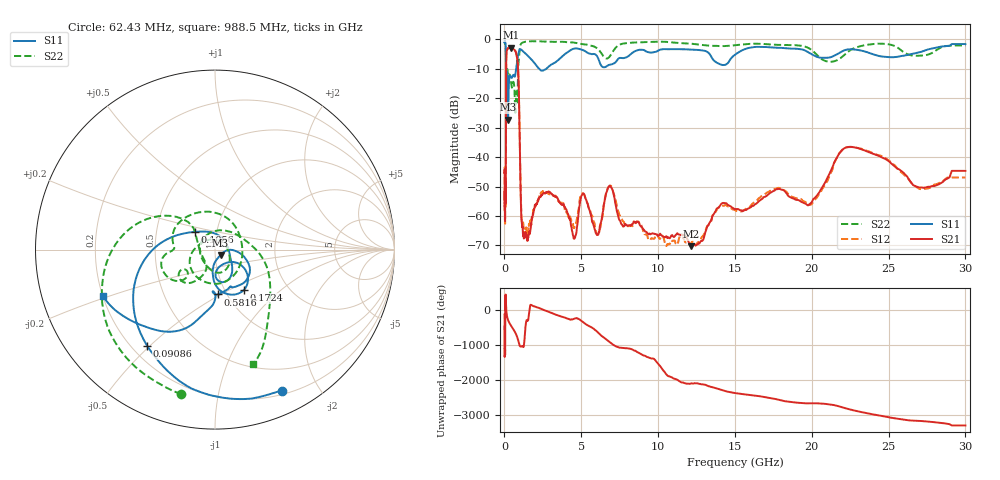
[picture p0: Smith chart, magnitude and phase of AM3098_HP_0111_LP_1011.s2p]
! Date/Time: Thu, Feb 28, 2019 8:39 AM
! Network Analyzer: Agilent Technologies E8364B Rev: A.07.50.67
! Sweep from 0.010 to 30.000 GHz, 1601 Points, Sweep Type: LOG
! Power Supply: 5.022 V, 0.002 A
# Hz S DB R 50
!freq MagS11 AngS11 MagS21 AngS21 MagS12 AngS12 MagS22 AngS22
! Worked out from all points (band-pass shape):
!   1601 points, 10 MHz to 30 GHz, reference 50 ohm
!   highest |S21| = -2.83 dB at 409.7 MHz (marker M1); lowest = -70.2 dB at 12.13 GHz (marker M2)
!   |S21| within 3 dB of the highest: 122.1 MHz to 807.7 MHz (685.6 MHz wide, 147 % of centre)
!   lowest |S11| = -27.2 dB at 238.7 MHz (marker M3), VSWR 1.09, Z = 53.1 - j3.22 ohm
!   |S11| at or under -10 dB: 102.2 MHz to 756.9 MHz (654.8 MHz wide, 152 % of centre); 2.273 GHz to 2.717 GHz (444.2 MHz wide, 17.8 % of centre)
!   |S22| runs from -24.9 to -0.6 dB; largest |S21 - S12| = 0.012
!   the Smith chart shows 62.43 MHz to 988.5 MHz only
!   S11 on the Smith chart (normalised r, x): 62.43 MHz: 0.24, -1.56; 90.86 MHz: 0.26, -0.49; 105.6 MHz: 0.78, +0.16; 172.4 MHz: 1.22, -0.60; 581.6 MHz: 0.91, -0.48; 988.5 MHz: 0.20, -0.19
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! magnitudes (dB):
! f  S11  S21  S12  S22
! 10 MHz  -0.4  -45.3  -43.3  -0.6
! 38.04 MHz  -0.4  -61.4  -60.0  -0.9
! 62.43 MHz  -1.2  -51.6  -51.8  -1.7
! 90.86 MHz  -3.7  -43.3  -42.2  -4.0
! 105.6 MHz  -16.5  -14.2  -14.2  -20.3
! 144.7 MHz  -19.7  -4.0  -4.0  -14.1
! 172.4 MHz  -11.2  -3.6  -3.5  -10.5
! 238.7 MHz  -27.2  -3.0  -2.9  -12.4
! 409.7 MHz  -12.6  -2.8  -2.8  -13.6
! 550.5 MHz  -12.3  -3.2  -3.2  -14.6
! 581.6 MHz  -12.0  -3.3  -3.2  -14.4
! 859.3 MHz  -6.3  -8.1  -8.1  -17.6
! 988.5 MHz  -3.4  -32.6  -32.7  -3.4
! 1.104 GHz  -3.5  -60.3  -59.5  -1.3
! 1.238 GHz  -4.2  -67.0  -63.8  -1.0
! 2.084 GHz  -8.9  -56.0  -55.9  -0.6
! 4.548 GHz  -3.1  -67.7  -63.9  -1.1
! 6.855 GHz  -8.6  -49.6  -49.7  -5.8
! 7.926 GHz  -6.1  -63.0  -63.4  -1.2
! 12.13 GHz  -3.5  -70.2  -69.4  -1.4
! 22.56 GHz  -3.4  -36.5  -36.6  -3.5
! 30 GHz  -1.6  -44.7  -46.9  -2.0
